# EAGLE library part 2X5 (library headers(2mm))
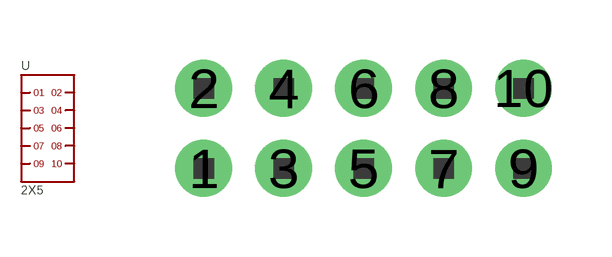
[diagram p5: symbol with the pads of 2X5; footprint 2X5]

Designator prefix -

## 2X5  [2X5]
1  1
2  2
3  3
4  4
5  5
6  6
7  7
8  8
9  9
10  10

## Footprint 2X5 (pad centres in mm)
drill 0.8 pad 1.422: 1 -4,-1; 2 -4,1; 3 -2,-1; 4 -2,1; 5 0,-1; 6 0,1; 7 2,-1; 8 2,1; 9 4,-1; 10 4,1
